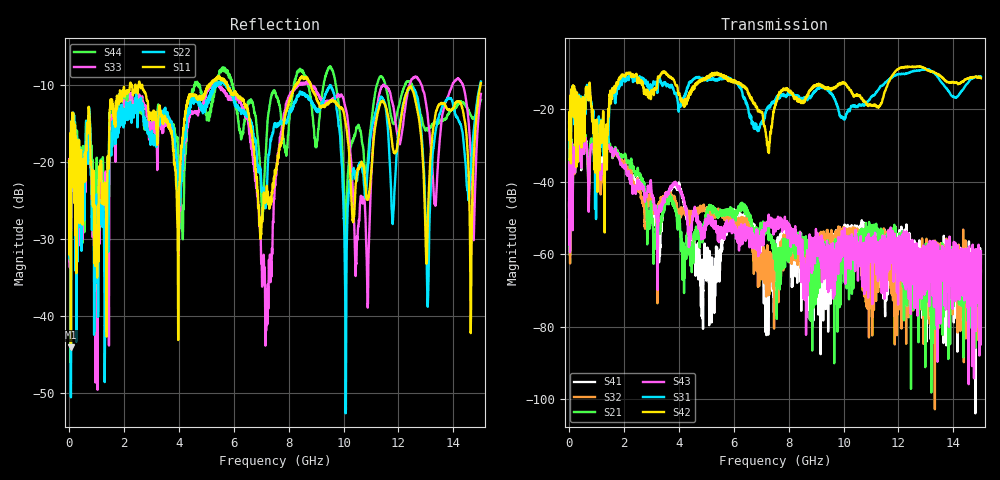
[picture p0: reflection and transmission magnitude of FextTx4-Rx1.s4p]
! FILE: N:\QM 2007\Prüfprotokolle\Highspeed\Konfektionierte Ltg\L45593-D106\D30\8216\0002\Fext\FextTx4-Rx1.s4p
# MHz S RI R 50.00
! FREQ  S11  S12  S13  S14
!  S21  S22  S23  S24
!  S31  S32  S33  S34
!  S41  S42  S43  S44
!  REAL  IMAG  REAL  IMAG  REAL  IMAG  REAL  IMAG
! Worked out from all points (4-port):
!   2999 points, 10 MHz to 15 GHz, reference 50 ohm
!   strongest paths, dB at 10 MHz, 3.755 GHz, 7.505 GHz, 11.26 GHz, 15 GHz:
!     S42: -23.8, -11.5, -19.4, -19.6, -11.6
!     S31: -25.6, -13.5, -18.0, -14.8, -11.1
!     S43: -46.4, -41.5, -51.1, -67.5, -59.2
!     S21: -44.8, -45.6, -58.5, -53.0, -61.0
!     S32: -50.5, -44.7, -66.1, -57.4, -60.0
!     S41: -45.7, -41.9, -61.7, -60.2, -64.6
!   lowest |S11| = -44.1 dB at 75 MHz (marker M1), VSWR 1.01, Z = 49.4 - j0.0188 ohm
!   |S11| at or under -10 dB: 2.672 GHz to 5.106 GHz (2.434 GHz wide, 62.6 % of centre); 5.778 GHz to 8.262 GHz (2.484 GHz wide, 35.4 % of centre); 8.8 GHz to 14.98 GHz (6.182 GHz wide, 52 % of centre)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
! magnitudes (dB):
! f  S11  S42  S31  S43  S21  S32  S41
! 10 MHz  -19.8  -23.8  -25.6  -46.4  -44.8  -50.5  -45.7
! 75 MHz  -44.1  -35.0  -32.4  -47.1  -44.0  -44.0  -44.8
! 5.43 GHz  -9.1  -10.3  -11.8  -52.3  -48.6  -48.9  -63.0
! 7.205 GHz  -23.1  -28.7  -20.3  -51.2  -53.0  -63.4  -68.8
! 12.49 GHz  -10.5  -8.3  -9.7  -57.3  -65.6  -63.0  -64.4
! 13.06 GHz  -27.8  -9.4  -9.1  -64.5  -69.6  -66.0  -66.2
! 15 GHz  -9.7  -11.6  -11.1  -59.2  -61.0  -60.0  -64.6
